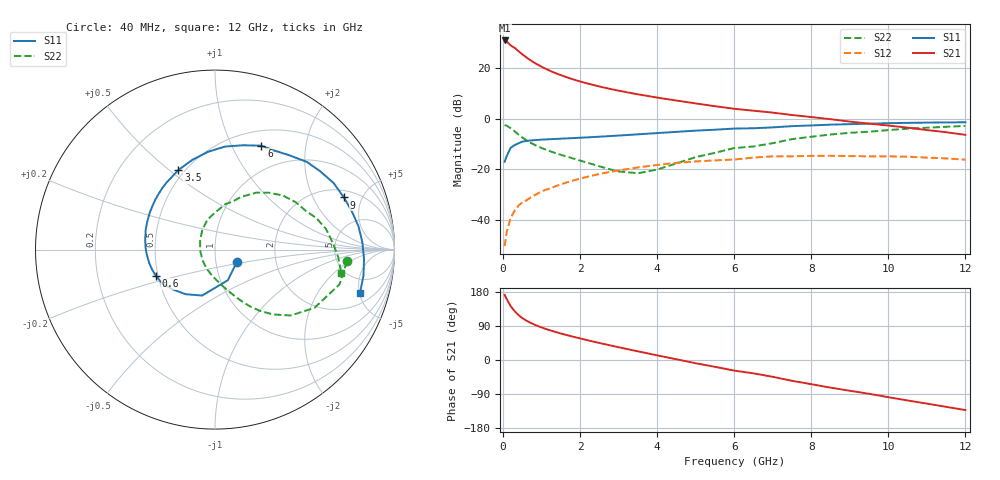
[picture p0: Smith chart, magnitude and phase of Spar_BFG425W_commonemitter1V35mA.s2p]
! Filename: 135bfg425.001
! BFG425W Field C1
! V1=8.936E-001V,V2=1.000E+000V, I1=5.768E-004A, I2=3.501E-002A
# GHz  S  MA  R 50
!  S11  S21  S12  S22
!Freq(GHz)  Mag  Ang  Mag  Ang  Mag  Ang  Mag  Ang
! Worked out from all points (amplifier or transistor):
!   44 points, 40 MHz to 12 GHz, reference 50 ohm
!   highest |S21| = 30.9 dB at 40 MHz (marker M1)
!   |S21| within 3 dB of that: start of sweep to 305.4 MHz
!   unconditionally stable (mu >= 1): start of sweep to 146.4 MHz; 570.2 MHz to end of sweep
!   at 700 MHz: K = 1.07, MAG = 25.7 dB, |S12| = -31.4 dB
!   at 2.4 GHz: K = 1.30, MAG = 14.4 dB, |S12| = -22.3 dB
!   at 12 GHz: K = 1.47, MAG = 0.8 dB, |S12| = -16.2 dB
!   S11 on the Smith chart (normalised r, x): 40 MHz: 1.26, -0.18; 600 MHz: 0.49, -0.16; 3.5 GHz: 0.46, +0.54; 6 GHz: 0.68, +1.31; 9 GHz: 2.44, +3.55; 12 GHz: 3.05, -5.08
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0.04  0.14 -29.8  35 172.1  0.003 68.4  0.738 -5.1
0.1  0.185 -67.3  33.02 159.7  0.006 76.4  0.72 -15.7
0.2  0.266 -105.7  27.93 141.5  0.011 69.7  0.642 -30.4
0.3  0.298 -123.5  24.98 128.9  0.015 65.6  0.559 -41.1
0.4  0.324 -137.0  21.5 118.7  0.019 63.4  0.484 -48.3
0.5  0.35 -147.9  18.61 110.6  0.022 61.9  0.423 -53.8
0.6  0.36 -156.0  16.29 104.2  0.024 61.1  0.376 -57.9
0.7  0.368 -162.6  14.38 98.8  0.027 60.4  0.338 -61.3
0.8  0.374 -168.3  12.87 94.0  0.03 59.9  0.307 -64.2
1.1  0.387 178.2  9.688 82.3  0.039 58.0  0.245 -71.7
1.3  0.394 171.0  8.275 75.8  0.044 56.4  0.215 -76.5
1.6  0.404 161.5  6.774 67.2  0.053 53.5  0.182 -83.8
2.2  0.425 145.0  4.914 52.0  0.071 46.2  0.133 -102.2
2.8  0.452 130.3  3.827 38.1  0.089 37.7  0.098 -129.2
3.5  0.488 114.7  3.013 22.8  0.108 27.0  0.083 -177.1
4.5  0.546 94.2  2.271 1.9  0.133 10.8  0.13 123.1
6  0.634 66.0  1.56 -28.0  0.155 -14.1  0.261 76.9
6.5  0.643 59.1  1.43 -35.2  0.169 -18.8  0.281 70.6
8.5  0.758 29.3  0.971 -73.0  0.184 -54.3  0.484 38.4
9  0.775 22.0  0.871 -81.1  0.181 -62.0  0.522 30.3
10.5  0.822 2.8  0.661 -106.8  0.176 -86.8  0.63 10.4
12  0.843 -16.6  0.476 -132.1  0.154 -113.8  0.716 -10.7
